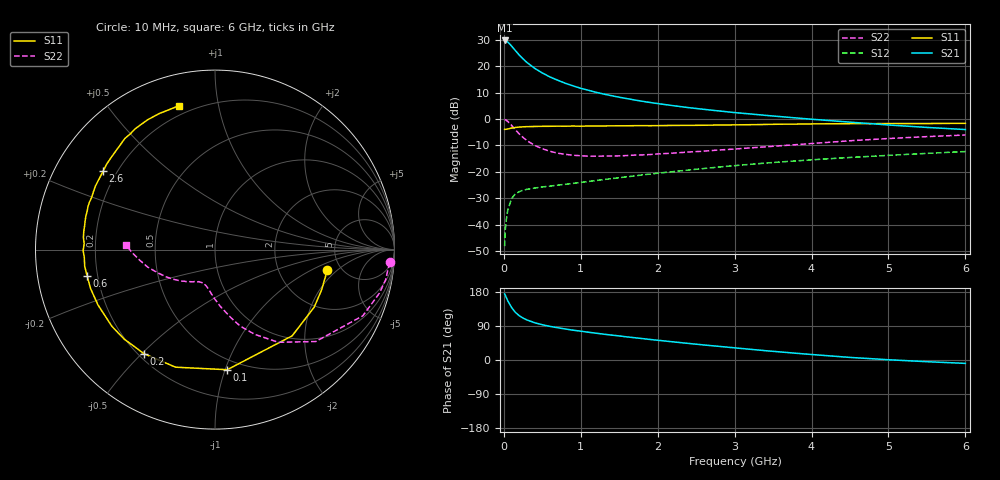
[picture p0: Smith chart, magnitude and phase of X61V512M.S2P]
! SIEMENS Small Signal Semiconductors
! BFP193W
! Si NPN RF Bipolar Junction Transistor in SOT343
! VCE = 1.5 V  IC = 12 mA
! Common Emitter S-Parameters:  April 1994
# GHz  S  MA  R  50
!  f  S11  S21  S12  S22
! GHz  MAG  ANG  MAG  ANG  MAG  ANG  MAG  ANG
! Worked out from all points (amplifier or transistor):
!   40 points, 10 MHz to 6 GHz, reference 50 ohm
!   highest |S21| = 29.7 dB at 10 MHz (marker M1)
!   |S21| within 3 dB of that: start of sweep to 126.2 MHz
!   unconditionally stable (mu >= 1): 1.159 GHz to 4.239 GHz
!   at 200 MHz: K = 0.26, MSG = 25.9 dB, |S12| = -27.6 dB
!   at 1.5 GHz: K = 1.10, MAG = 13.3 dB, |S12| = -22.2 dB
!   at 6 GHz: K = 0.94, MSG = 4.2 dB, |S12| = -12.3 dB
!   S11 on the Smith chart (normalised r, x): 10 MHz: 3.92, -1.47; 100 MHz: 0.42, -1.02; 200 MHz: 0.22, -0.51; 600 MHz: 0.16, -0.10; 2.6 GHz: 0.15, +0.31; 6 GHz: 0.15, +0.77
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0.01  0.6363 -10.1  30.71 174.4  0.0039 85.7  0.9757 -4.2
0.02  0.635 -20.5  30.7 170.3  0.0083 80.0  0.9654 -10.1
0.03  0.6391 -30.1  30.19 165.7  0.0118 78.7  0.9473 -14.9
0.05  0.6447 -48.2  28.79 156.7  0.0184 69.5  0.9025 -24.1
0.1  0.6727 -84.2  24.14 138.8  0.031 54.9  0.7597 -42.4
0.15  0.6909 -108.5  19.77 125.7  0.0383 44.9  0.6251 -55.7
0.2  0.7021 -124.3  16.28 117.0  0.0419 39.5  0.5214 -64.9
0.25  0.7103 -135.4  13.76 110.6  0.0449 35.8  0.4483 -71.8
0.3  0.7161 -143.4  11.76 105.7  0.0465 33.7  0.3891 -76.9
0.4  0.7212 -154.7  9.134 98.4  0.0492 32.2  0.3167 -84.8
0.5  0.7264 -162.6  7.441 93.0  0.0516 32.1  0.2731 -90.6
0.6  0.7274 -168.2  6.248 88.7  0.0536 33.0  0.2443 -95.2
0.8  0.7296 -176.5  4.746 81.8  0.0579 35.7  0.2138 -101.8
1.1  0.7363 174.7  3.494 73.3  0.0655 39.6  0.1978 -109.3
1.3  0.7385 169.7  2.961 68.1  0.0712 41.8  0.1981 -113.2
1.6  0.7436 163.3  2.431 61.0  0.0804 44.5  0.203 -118.0
2.2  0.7546 152.0  1.789 47.9  0.1006 47.0  0.2257 -127.7
2.6  0.7614 145.0  1.523 39.7  0.1153 47.3  0.2457 -134.3
3.2  0.7793 135.1  1.246 28.4  0.1384 46.0  0.2834 -144.1
4.5  0.8149 117.5  0.871 6.8  0.1867 40.0  0.3871 -165.4
5.5  0.8203 108.2  0.692 -4.5  0.2231 34.4  0.4634 -178.1
6  0.827 103.9  0.631 -8.9  0.2419 31.9  0.4974 176.9
